(* Logix 5000 AddOnInstructionDefinition export Banner_Thickness_AOI; software revision 30.00 *)

TYPE Banner_Thickness_Tags :   // Tags needed to calculate the thickness of a part using the Banner Thickness AOI.
STRUCT
   CF1 : REAL;   // Conversion Factor for Sensor 1
   CF2 : REAL;   // Conversion Factor for Sensor 2
   Zero1 : REAL;   // Calibrated zero value for taught target
   Zero2 : REAL;   // Calibrated zero value for taught target
   Nominal_Value : REAL;   // Nominal Value of taught target in real units (mm or inches)
   Thickness_Value : REAL;   // Current thickness of the target
   Teach_Request : BOOL;   // Request the current target to be taught
   State : INT;   // 0 = System has yet to be taught. 1 = System taught.
END_STRUCT
END_TYPE

ADD_ON_INSTRUCTION Banner_Thickness_AOI   (* revision 1.0, vendor Banner Engineering *)
// Calculate the thickness of an object.
VAR_INPUT
   Sensor1 : REAL; {required}   // Sensor 1 reading
   Sensor2 : REAL; {required}   // Sensor 2 reading
END_VAR
VAR_IN_OUT
   Thickness : Banner_Thickness_Tags; {required}   // UDT for Banner Thickness AOI.
        .CF1   // Conversion Factor for Sensor 1
        .CF2   // Conversion Factor for Sensor 2
        .ZERO1   // Calibrated zero value for target
        .ZERO2   // Calibrated zero value for target
        .NOMINAL_VALUE   // Nominal value of taught target in real units (mm or inches)
        .THICKNESS_VALUE   // Current thickness of target
        .TEACH_REQUEST   // Request the current target to be taught
        .STATE   // 0 = System has yet to be taught, 1 = System taught
END_VAR

ROUTINE Logic   (* ladder *)
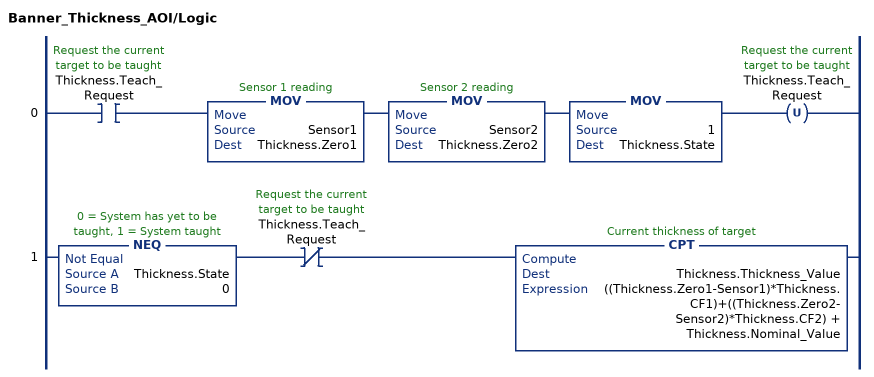
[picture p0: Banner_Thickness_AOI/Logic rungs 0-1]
   0: XIC(Thickness.Teach_Request)MOV(Sensor1,Thickness.Zero1)MOV(Sensor2,Thickness.Zero2)MOV(1,Thickness.State)OTU(Thickness.Teach_Request);
   1: NEQ(Thickness.State,0)XIO(Thickness.Teach_Request)CPT(Thickness.Thickness_Value,((Thickness.Zero1-Sensor1)*Thickness.CF1)+((Thickness.Zero2-Sensor2)*Thickness.CF2) + Thickness.Nominal_Value);
END_ROUTINE
END_ADD_ON_INSTRUCTION
